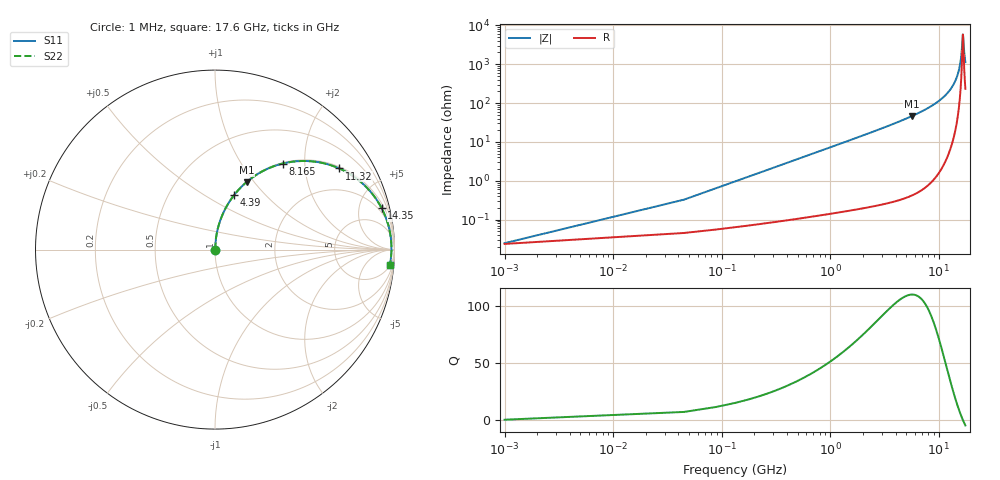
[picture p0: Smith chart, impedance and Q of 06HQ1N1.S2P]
! Coilcraft 0604HQ-1N1 Chip Inductor
! 15 August 2002
# MHZ S MA R 50
!Freq  MagS11  AngS11  MagS21  AngS21  MagS12  AngS12  MagS22  AngS22
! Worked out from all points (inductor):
!   402 points, 1 MHz to 17.6 GHz, reference 50 ohm
!   read as one part in series: L = 1.15 nH near 88.78 MHz
!   highest Q = 110 at 5.619 GHz (marker M1), where L = 1.3 nH
!   self-resonance near 16.68 GHz
!   S11 on the Smith chart (normalised r, x): 1 MHz: 1.00, +0.00; 4.39 GHz: 1.01, +0.68; 8.165 GHz: 1.02, +1.55; 11.32 GHz: 1.06, +3.03; 14.35 GHz: 1.45, +7.91; 17.6 GHz: 6, -22
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1  0.0002488 16.9  0.9998 -0.0  0.9998 -0.0  0.0002488 16.9
132.67  0.009602 85.6  0.9993 -0.5  0.9993 -0.5  0.009602 85.6
176.56  0.01277 86.1  0.9992 -0.7  0.9992 -0.7  0.01277 86.1
308.23  0.02227 86.5  0.9989 -1.3  0.9989 -1.3  0.02227 86.5
527.68  0.03811 86.2  0.9982 -2.2  0.9982 -2.2  0.03811 86.2
1405.48  0.1016 83.2  0.9932 -5.8  0.9932 -5.8  0.1016 83.2
2941.63  0.2138 77.0  0.9745 -12.3  0.9745 -12.3  0.2138 77.0
4390  0.3216 70.7  0.9438 -18.8  0.9438 -18.8  0.3216 70.7
5618.92  0.4149 65.0  0.9061 -24.5  0.9061 -24.5  0.4149 65.0
5882.26  0.435 63.7  0.8965 -25.8  0.8965 -25.8  0.435 63.7
8164.54  0.6096 51.8  0.7863 -37.6  0.7863 -37.6  0.6096 51.8
8822.89  0.6588 48.1  0.7449 -41.2  0.7449 -41.2  0.6588 48.1
11324.62  0.8274 33.1  0.5462 -55.8  0.5462 -55.8  0.8274 33.1
11763.52  0.8523 30.3  0.5052 -58.4  0.5052 -58.4  0.8523 30.3
14353.03  0.9567 13.9  0.2414 -72.8  0.2414 -72.8  0.9567 13.9
14704.15  0.9647 11.8  0.2045 -74.2  0.2045 -74.2  0.9647 11.8
15889.18  0.9809 4.6  0.08244 -74.3  0.08244 -74.3  0.9809 4.6
16240.3  0.9827 2.6  0.04826 -67.7  0.04826 -67.7  0.9827 2.6
16679.2  0.9832 0.1  0.01693 -6.7  0.01693 -6.7  0.9832 0.1
16810.87  0.983 -0.6  0.02011 31.8  0.02011 31.8  0.983 -0.6
17205.88  0.9813 -2.8  0.05159 67.4  0.05159 67.4  0.9813 -2.8
17600  0.9784 -4.9  0.08702 73.2  0.08702 73.2  0.9784 -4.9
